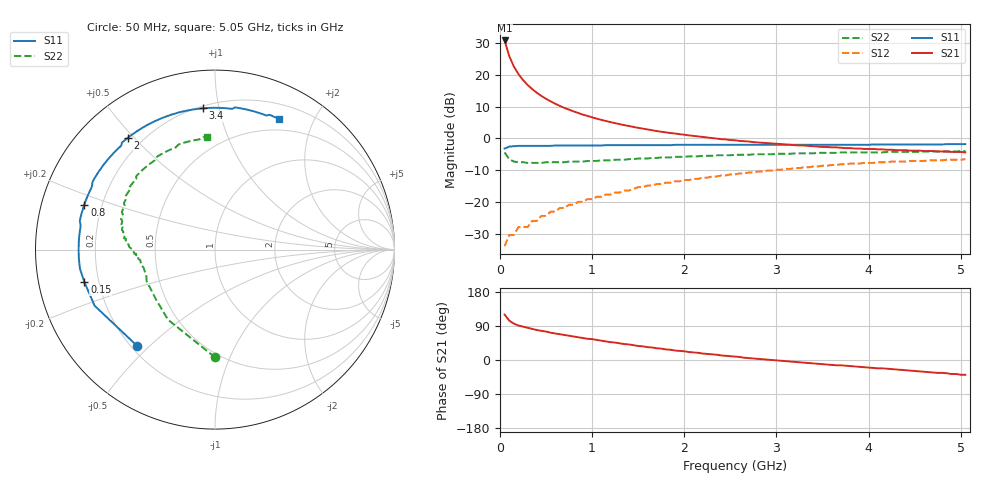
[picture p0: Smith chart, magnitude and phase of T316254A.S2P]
!AT-31625
!S-PARAMETERS at Vce=3.6 V  Ic=50 mA.  LAST UPDATED 08-05-96
# ghz s ma r 50
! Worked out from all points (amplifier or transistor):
!   101 points, 50 MHz to 5.05 GHz, reference 50 ohm
!   highest |S21| = 30.8 dB at 50 MHz (marker M1)
!   |S21| within 3 dB of that: start of sweep to 80.49 MHz
!   unconditionally stable (mu >= 1): 489.3 MHz to 524.9 MHz; 570.9 MHz to 646.2 MHz; 652 MHz to 1.445 GHz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
!   at 850 MHz: K = 1.02, MAG = 13.1 dB, |S12| = -20.0 dB
!   at 2.55 GHz: K = 0.93, MSG = 5.4 dB, |S12| = -11.4 dB
!   at 5.05 GHz: K = 0.95, MSG = 1.1 dB, |S12| = -6.6 dB
!   S11 on the Smith chart (normalised r, x): 50 MHz: 0.22, -0.46; 150 MHz: 0.14, -0.12; 800 MHz: 0.13, +0.16; 2 GHz: 0.14, +0.48; 3.4 GHz: 0.21, +0.89; 5.05 GHz: 0.36, +1.54
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0.05  0.69 -129.0  34.76 120.0  0.02 43.0  0.6 -90.0
0.1  0.74 -155.0  19.73 104.0  0.03 38.0  0.47 -124.0
0.15  0.75 -166.0  13.53 96.0  0.03 40.0  0.43 -140.0
0.2  0.76 -172.0  10.27 91.0  0.04 44.0  0.42 -149.0
0.25  0.76 -176.0  8.27 88.0  0.04 47.0  0.42 -155.0
0.3  0.76 -179.0  6.91 85.0  0.04 50.0  0.41 -159.0
0.35  0.76 178.0  5.95 82.0  0.05 53.0  0.41 -162.0
0.4  0.76 176.0  5.21 79.0  0.05 55.0  0.41 -164.0
0.45  0.76 174.0  4.64 77.0  0.06 56.0  0.41 -166.0
0.5  0.76 172.0  4.19 75.0  0.06 57.0  0.42 -168.0
0.55  0.76 170.0  3.81 72.0  0.07 58.0  0.42 -169.0
0.65  0.77 166.0  3.23 68.0  0.08 60.0  0.42 -171.0
0.8  0.77 161.0  2.65 62.0  0.09 60.0  0.43 -173.0
0.9  0.77 158.0  2.36 58.0  0.1 60.0  0.43 -175.0
1.2  0.78 150.0  1.8 47.0  0.13 58.0  0.45 -178.0
1.5  0.78 142.0  1.46 37.0  0.17 55.0  0.48 178.0
1.75  0.78 135.0  1.27 30.0  0.19 52.0  0.5 175.0
2  0.79 128.0  1.14 23.0  0.22 48.0  0.51 171.0
2.55  0.79 115.0  0.93 9.0  0.27 39.0  0.55 162.0
3.4  0.79 95.0  0.75 -9.0  0.36 23.0  0.58 145.0
4.25  0.8 78.0  0.66 -24.0  0.43 4.0  0.61 121.0
5.05  0.81 64.0  0.6 -39.0  0.47 -13.0  0.63 94.0
